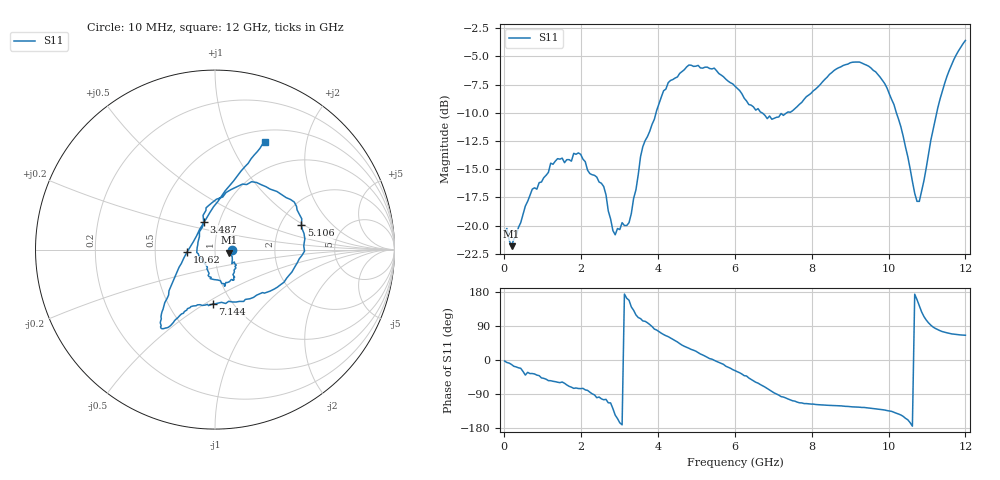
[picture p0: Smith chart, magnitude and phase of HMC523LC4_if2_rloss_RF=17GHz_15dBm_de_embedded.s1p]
!Hittite Microwave Corporation
!20 Alpha Rd
!Chelmsford, MA 01824
!Tel: 978-250-3343
!Fax: 978-250-3373
!Device: HMC523LC4, 0.01-12 GHz, GaAs MMIC Double-Balanced Mixer
!Misc: IF2 Return Loss with RF=17GHz at 15 dBm, Room
# MHZ S MA R 50
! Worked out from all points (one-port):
!   201 points, 10 MHz to 12 GHz, reference 50 ohm
!   lowest |S11| = -21.8 dB at 189.8 MHz (marker M1), VSWR 1.18, Z = 58.6 - j1.97 ohm
!   |S11| at or under -10 dB: start of sweep to 3.951 GHz; 6.706 GHz to 7.351 GHz (644.8 MHz wide, 9.17 % of centre); 10.2 GHz to 11.25 GHz (1.049 GHz wide, 9.78 % of centre)
!   S11 on the Smith chart (normalised r, x): 10 MHz: 1.21, -0.01; 3.487 GHz: 0.84, +0.27; 5.106 GHz: 2.61, +0.95; 7.144 GHz: 0.81, -0.54; 10.62 GHz: 0.73, -0.02; 12 GHz: 0.63, +1.36
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10  0.094 -2.7
189.85  0.081 -11.9
729.4  0.145 -35.7
1508.75  0.199 -58.1
1988.35  0.207 -75.5
2587.85  0.149 -104.9
2827.65  0.095 -128.1
3007.5  0.096 -165.8
3247.3  0.103 157.7
3487.1  0.168 112.0
3607  0.224 103.1
4146.55  0.396 67.2
4506.25  0.456 47.6
4806  0.515 30.9
5105.75  0.5 15.8
5465.45  0.499 -0.9
6005  0.415 -28.0
6844.3  0.298 -75.2
7144.05  0.303 -92.6
7503.75  0.323 -107.6
9002.5  0.527 -123.2
9901.75  0.426 -132.1
10141.55  0.344 -138.2
10501.25  0.202 -157.8
10621.15  0.157 -174.6
10801  0.128 143.4
11340.55  0.364 77.3
12000  0.662 65.3
